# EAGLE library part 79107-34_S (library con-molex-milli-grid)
RECEPTACAL
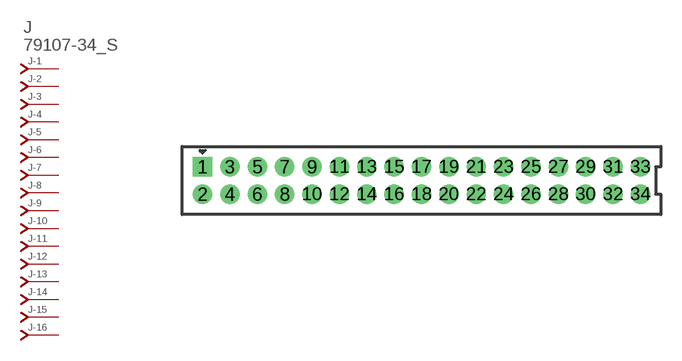
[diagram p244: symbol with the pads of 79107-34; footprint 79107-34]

Designator prefix J; gates -1=J-NV -2=J-N -3=J-N -4=J-N -5=J-N -6=J-N -7=J-N -8=J-N -9=J-N -10=J-N -11=J-N -12=J-N -13=J-N -14=J-N -15=J-N -16=J-N -17=J-N -18=J-N -19=J-N -20=J-N -21=J-N -22=J-N -23=J-N -24=J-N -25=J-N -26=J-N -27=J-N -28=J-N -29=J-N -30=J-N -31=J-N -32=J-N -33=J-N -34=J-N

## 79107-34_S  [79107-34]
1  -1:J  pas
2  -2:J  pas
3  -3:J  pas
4  -4:J  pas
5  -5:J  pas
6  -6:J  pas
7  -7:J  pas
8  -8:J  pas
9  -9:J  pas
10  -10:J  pas
11  -11:J  pas
12  -12:J  pas
13  -13:J  pas
14  -14:J  pas
15  -15:J  pas
16  -16:J  pas
17  -17:J  pas
18  -18:J  pas
19  -19:J  pas
20  -20:J  pas
21  -21:J  pas
22  -22:J  pas
23  -23:J  pas
24  -24:J  pas
25  -25:J  pas
26  -26:J  pas
27  -27:J  pas
28  -28:J  pas
29  -29:J  pas
30  -30:J  pas
31  -31:J  pas
32  -32:J  pas
33  -33:J  pas
34  -34:J  pas

## Footprint 79107-34 (pad centres in mm)
RECEPTACAL Dual Row, Vertical, Through-Hole
drill 0.914 square: 1 -16,1
drill 0.914: 2 -16,-1; 3 -14,1; 4 -14,-1; 5 -12,1; 6 -12,-1; 7 -10,1; 8 -10,-1; 9 -8,1; 10 -8,-1; 11 -6,1; 12 -6,-1; 13 -4,1; 14 -4,-1; 15 -2,1; 16 -2,-1; 17 0,1; 18 0,-1; 19 2,1; 20 2,-1; 21 4,1; 22 4,-1; 23 6,1; 24 6,-1; 25 8,1; 26 8,-1; 27 10,1; 28 10,-1; 29 12,1; 30 12,-1; 31 14,1; 32 14,-1; 33 16,1; 34 16,-1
